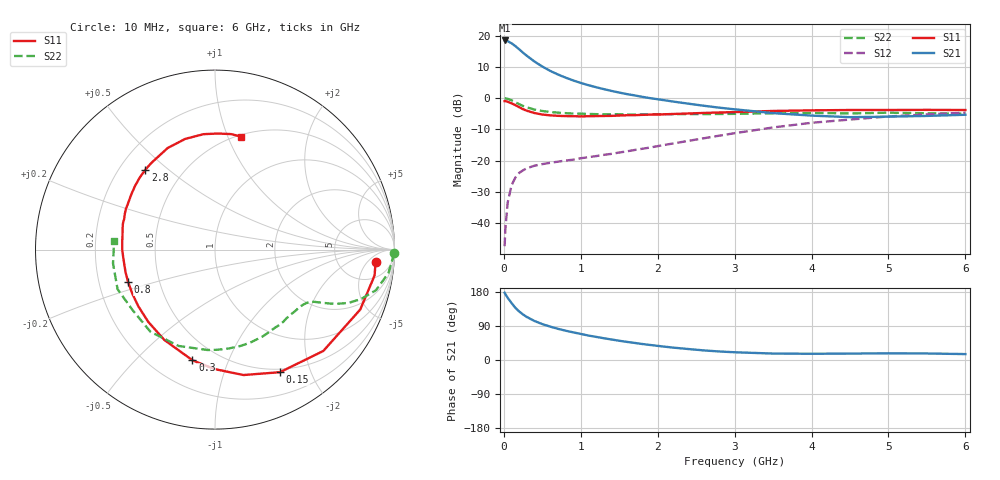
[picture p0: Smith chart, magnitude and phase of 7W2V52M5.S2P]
! Infineon Technologies  Discrete & RF Semiconductors
! BFS17W
! Si NPN RF Bipolar Junction Transistor in SOT323
! VCE = 2.5 V  IC = 2.5 mA
! Common Emitter S-Parameters:  August  1999
# GHz  S  MA  R  50
!  f  S11  S21  S12  S22
! GHz  MAG  ANG  MAG  ANG  MAG  ANG  MAG  ANG
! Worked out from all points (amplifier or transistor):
!   36 points, 10 MHz to 6 GHz, reference 50 ohm
!   highest |S21| = 18.5 dB at 10 MHz (marker M1)
!   |S21| within 3 dB of that: start of sweep to 207.6 MHz
!   unconditionally stable (mu >= 1): 745.3 MHz to end of sweep
!   at 250 MHz: K = 0.41, MSG = 18.8 dB, |S12| = -23.1 dB
!   at 1.4 GHz: K = 1.32, MAG = 6.7 dB, |S12| = -17.8 dB
!   at 6 GHz: K = 1.10, MAG = -2.3 dB, |S12| = -4.6 dB
!   S11 on the Smith chart (normalised r, x): 10 MHz: 12, -9; 150 MHz: 0.46, -1.56; 300 MHz: 0.37, -0.75; 800 MHz: 0.33, -0.16; 2.8 GHz: 0.31, +0.42; 6 GHz: 0.52, +1.12
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0.01  0.8974 -4.4  8.369 177.5  0.0043 83.2  0.9978 -1.1
0.02  0.9007 -9.2  8.344 173.8  0.0082 88.2  0.9905 -3.1
0.05  0.8755 -22.4  8.157 164.2  0.0215 77.6  0.9751 -7.7
0.1  0.8265 -43.1  7.543 150.3  0.0404 67.7  0.9256 -14.1
0.15  0.773 -62.1  6.794 137.8  0.0539 58.8  0.8593 -18.7
0.2  0.7166 -77.2  6.039 128.0  0.0639 53.1  0.8003 -21.8
0.25  0.6656 -90.2  5.327 120.1  0.0702 48.0  0.7502 -23.7
0.3  0.6293 -101.5  4.749 113.4  0.0759 45.4  0.7125 -25.0
0.4  0.5771 -119.3  3.842 102.8  0.0833 41.9  0.6564 -26.7
0.5  0.548 -132.8  3.208 94.8  0.0882 40.7  0.6236 -27.8
0.6  0.5313 -143.5  2.739 88.2  0.0924 40.6  0.6012 -29.1
0.7  0.522 -152.1  2.4 82.5  0.0964 41.6  0.5871 -30.7
0.8  0.5168 -159.4  2.137 77.5  0.1005 42.4  0.5762 -32.6
1.1  0.5138 -176.1  1.612 64.5  0.114 46.8  0.5595 -38.9
1.3  0.5191 174.8  1.394 57.4  0.124 50.2  0.5522 -44.0
1.6  0.5331 164.3  1.161 47.8  0.1412 54.2  0.549 -51.9
2.2  0.5583 146.8  0.883 32.7  0.1887 60.1  0.5542 -69.6
2.8  0.5902 131.2  0.705 22.5  0.2512 61.1  0.5582 -88.4
3.5  0.6244 115.0  0.577 17.0  0.3404 57.6  0.5739 -110.7
4.5  0.6463 95.6  0.497 16.9  0.4548 45.8  0.5697 -143.9
5.5  0.6497 82.1  0.52 17.2  0.5499 33.5  0.5734 -172.3
6  0.6463 76.8  0.543 15.6  0.5867 27.6  0.564 175.2
